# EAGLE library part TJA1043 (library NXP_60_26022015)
High-speed CAN transceiver The TJA1043 is a high-speed CAN transceiver that provides an interface between a Controller Area Network (CAN) protocol controller and the physical two-wire CAN bus. The transceiver is designed for high-speed (up to 1 Mbit/s) CAN applications in the automotive industry, providing differential transmit and receive capability to (a microcontroller with) a CAN protocol controller. The TJA1043 belongs to the third generation of high-speed CAN transceivers from NXP Semiconductors, offering significant improvements over first- and second-generation devices such as the TJA1041A. It offers improved ElectroMagnetic Compatibility (EMC) and ElectroMagnetic Discharge (ESD) performance, very low power consumption, and passive behavior when the supply voltage is turned off. Advanced features include: Low-power management controls the power supply throughout the node while supporting local and remote wake-up with wake-up source recognition Several protection and diagnostic functions including bus line short-circuit detection and battery connection detection Can be interfaced directly to microcontrollers with supply voltages from 3 V to 5 V These features make the TJA1043 the ideal choice for high speed CAN networks containing nodes that need to be available all times, even when the internal VIO and VCC supplies are switched off. AAL Eindhoven MK
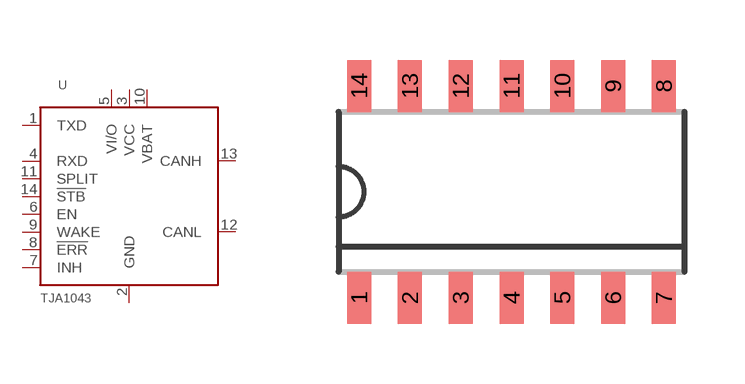
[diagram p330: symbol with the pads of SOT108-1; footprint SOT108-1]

Designator prefix U

## TJA1043T  [SOT108-1]
1  TXD  out
2  GND  pwr
3  VCC  pwr
4  RXD
5  VI/O  pwr
6  EN  in
7  INH  in
8  !ERR  out
9  WAKE  in
10  VBAT  pwr
11  SPLIT  pwr
12  CANL
13  CANH
14  !STB  in

## Footprint SOT108-1 (pad centres in mm)
SOT108-1 SO14: plastic small outline package; 14 leads; body width 3.9 mm; body thickness 1.47 mm JEDEC: MS-012 IEC: --
smd 0.6 x 1.3: 1 -3.81,-2.65; 2 -2.54,-2.65; 3 -1.27,-2.65; 4 0,-2.65; 5 1.27,-2.65; 6 2.54,-2.65; 7 3.81,-2.65; 8 3.81,2.65; 9 2.54,2.65; 10 1.27,2.65; 11 0,2.65; 12 -1.27,2.65; 13 -2.54,2.65; 14 -3.81,2.65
